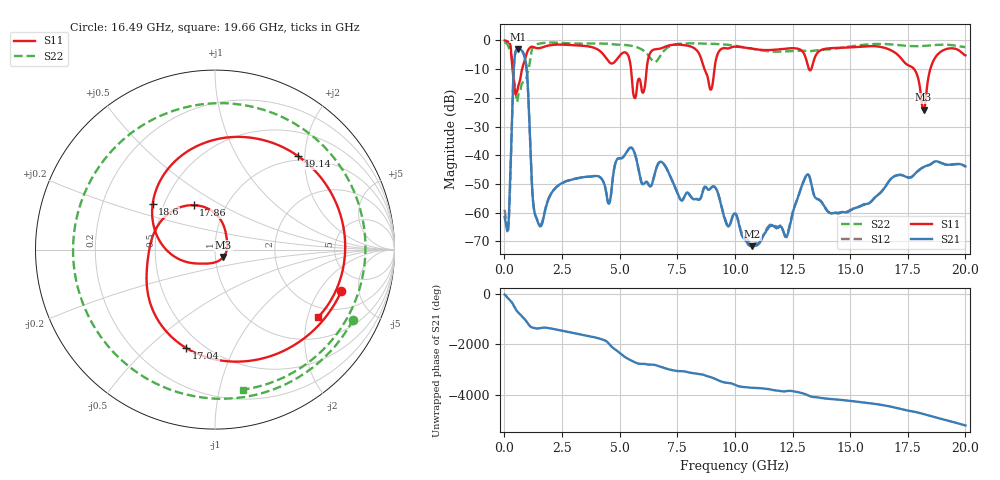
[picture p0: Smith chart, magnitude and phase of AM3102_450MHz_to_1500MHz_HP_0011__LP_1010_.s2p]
!Agilent Technologies,E8364B,MY43040894,A.07.50.67
!Agilent E8364B: A.07.50.67
!Date: Thursday, January 11, 2018 05:32:44
!Correction: S11(Full 2 Port(1,2))
!S21(Full 2 Port(1,2))
!S12(Full 2 Port(1,2))
!S22(Full 2 Port(1,2))
!S2P File: Measurements: S11, S21, S12, S22:
# Hz S  dB  R 50
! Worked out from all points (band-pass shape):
!   1601 points, 10 MHz to 20 GHz, reference 50 ohm
!   highest |S21| = -3.00 dB at 597.2 MHz (marker M1); lowest = -71.6 dB at 10.75 GHz (marker M2)
!   |S21| within 3 dB of the highest: 444.3 MHz to 885.8 MHz (441.5 MHz wide, 66.4 % of centre)
!   lowest |S11| = -24.1 dB at 18.19 GHz (marker M3), VSWR 1.13, Z = 54.7 - j4.54 ohm
!   |S11| at or under -10 dB: 5.493 GHz to 6.172 GHz (678.5 MHz wide, 11.6 % of centre); 8.679 GHz to 9.112 GHz (432.1 MHz wide, 4.86 % of centre); 17.77 GHz to 18.48 GHz (704.3 MHz wide, 3.89 % of centre)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
!   |S22| runs from -21.4 to -0.6 dB; largest |S21 - S12| = 0.0039
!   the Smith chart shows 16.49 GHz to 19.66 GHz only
!   S11 on the Smith chart (normalised r, x): 16.49 GHz: 3.21, -3.28; 17.04 GHz: 0.41, -0.67; 17.86 GHz: 0.70, +0.38; 18.6 GHz: 0.43, +0.27; 19.14 GHz: 0.92, +1.86; 19.66 GHz: 1.65, -2.34
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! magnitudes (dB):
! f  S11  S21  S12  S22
! 10 MHz  -0.1  -61.5  -59.0  -0.6
! 172.4 MHz  -0.6  -64.7  -65.1  -2.1
! 422.3 MHz  -15.2  -8.1  -8.1  -14.2
! 597.2 MHz  -16.1  -3.0  -3.0  -19.2
! 934.5 MHz  -5.5  -8.0  -8.0  -13.5
! 1.459 GHz  -2.8  -63.6  -63.0  -1.3
! 3.346 GHz  -1.9  -47.7  -47.7  -1.2
! 5.657 GHz  -20.1  -39.4  -39.4  -2.2
! 6.682 GHz  -3.0  -42.8  -42.8  -6.5
! 8.956 GHz  -17.2  -51.4  -51.4  -1.2
! 10.01 GHz  -2.2  -60.3  -60.2  -1.9
! 10.75 GHz  -3.0  -71.6  -71.0  -2.9
! 13.34 GHz  -9.4  -50.9  -50.9  -3.7
! 16.49 GHz  -2.6  -51.4  -51.3  -1.3
! 16.68 GHz  -3.1  -49.2  -49.0  -1.4
! 17.04 GHz  -4.9  -47.0  -46.9  -1.6
! 17.86 GHz  -11.2  -46.0  -46.1  -2.0
! 18.19 GHz  -24.1  -44.1  -44.1  -2.0
! 18.6 GHz  -7.3  -42.5  -42.5  -1.7
! 19.14 GHz  -3.1  -43.2  -43.3  -1.5
! 19.66 GHz  -3.3  -43.1  -43.0  -2.0
! 20 GHz  -5.2  -43.9  -43.9  -2.4
